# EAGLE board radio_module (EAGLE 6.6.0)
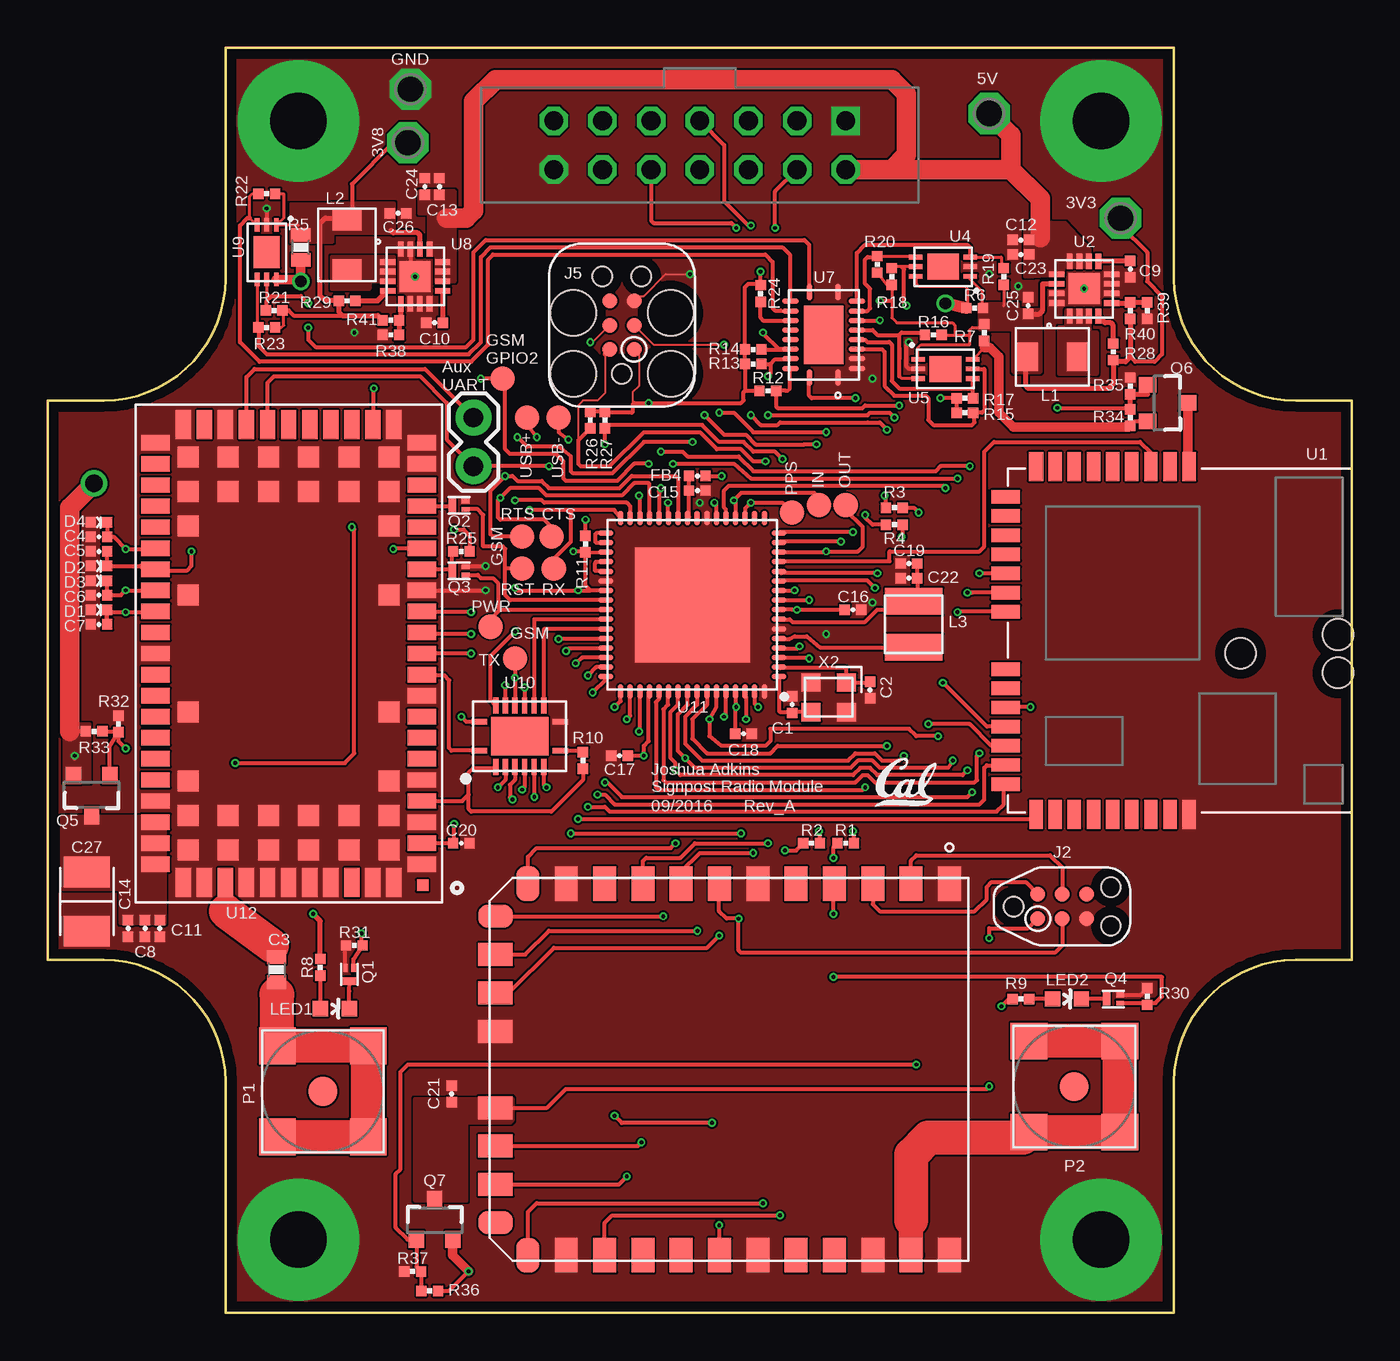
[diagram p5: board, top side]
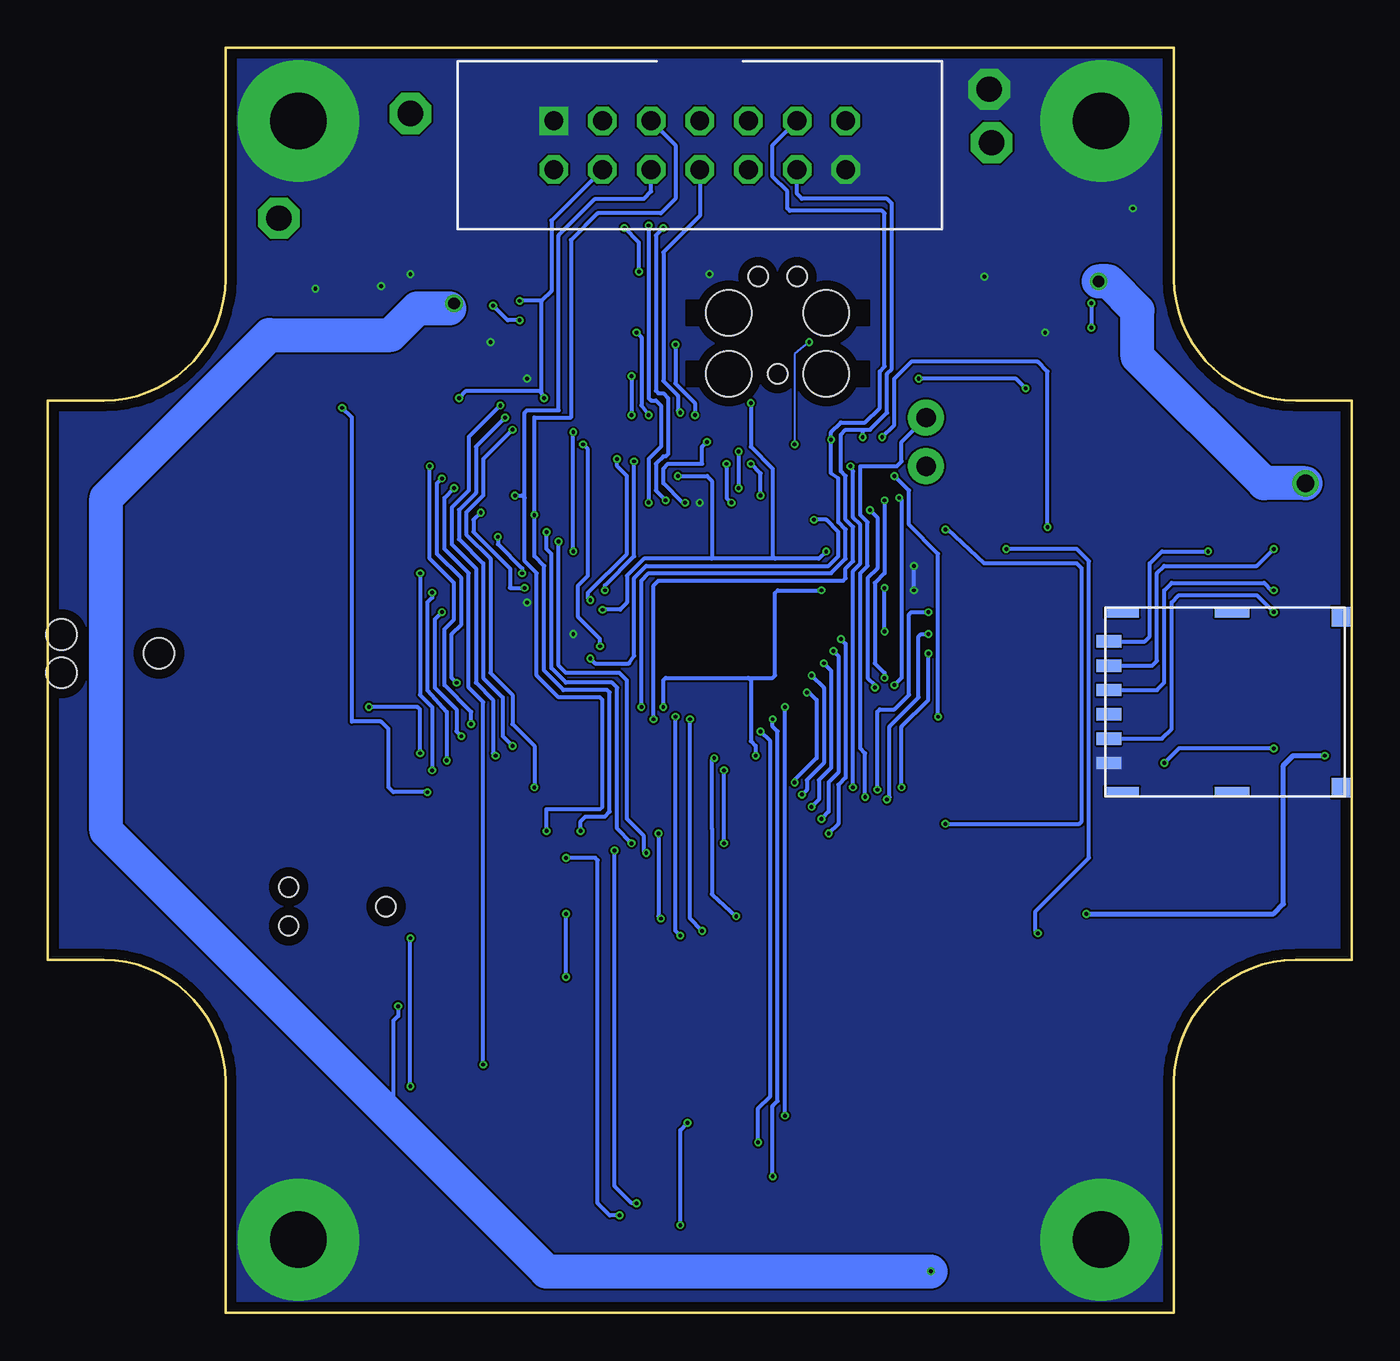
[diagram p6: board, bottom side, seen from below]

Size 68.07 x 66.04 mm. Coordinates in mm from the lower left corner, seen from the top.
Outline: 9.27,66.04 58.8,66.04 58.8,53.98 arc90 65.15,47.62 68.07,47.62 68.07,18.41 65.15,18.41 arc90 58.8,12.07 58.8,0 9.27,0 9.27,12.07 arc90 2.92,18.41 0,18.41 0,47.62 2.92,47.62 arc90 9.27,53.98 9.27,66.04
Copper layers (1*16): Top 0.0178mm / dielectric 59mil / Bottom 0.0178mm
Design rules "quickturn_co_kr_1oz *": minimum track width 4mil, minimum drill 0.200659375mm, track to track 4mil, track to pad 4mil, pad to pad 4mil, via to via 4mil, smd to smd 4mil, copper to edge 20mil, drill to drill 16mil, minimum pad ring 8mil, minimum via ring 4mil, stop-mask expansion 3mil, vias tented up to drill 50mil, thermal gap 10mil

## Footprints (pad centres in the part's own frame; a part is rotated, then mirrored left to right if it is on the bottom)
0402_CAP = smd 0.536 x 0.546: 1 -0.433,0; 2 0.433,0
0603_CAP = smd 0.7 x 1: 1 -0.65,0; 2 0.65,0
1210_CAP = smd 2.4 x 1.6: 1 0,1.55; 2 0,-1.55
0402_DIODE = smd 0.536 x 0.546: ANODE -0.433,0; CATHODE 0.433,0
MODULE_GENERIC = drill 0.991 square: 1 7.62,29.21 | drill 0.991 octagon: 2 7.62,26.67; 3 5.08,29.21; 4 5.08,26.67; 5 2.54,29.21; 6 2.54,26.67; 7 0,29.21; 8 0,26.67; 9 -2.54,29.21; 10 -2.54,26.67; 11 -5.08,29.21; 12 -5.08,26.67; 13 -7.62,29.21; 14 -7.62,26.67
TC2030-IDC-NL = smd 0.787 x 0.787: 1 -1.27,-0.635; 2 -1.27,0.635; 3 0,-0.635; 4 0,0.635; 5 1.27,-0.635; 6 1.27,0.635 | hole 1.016: -2.54,0; 2.54,1.016; 2.54,-1.016
WURTH_NANO_SIM = smd 0.65 x 1.3: C1 -1.905,6.07; C2 0.635,6.07; C3 1.905,6.07; C5 -3.175,6.07; C6 -0.635,6.07; C7 3.175,6.07 | smd 1.03 x 1: P$8 -4.465,-6.07; P$9 4.465,-6.07 | smd 0.48 x 1.8: P$10 -4.66,-0.35; P$11 4.66,-0.35; P$12 -4.66,5.4; P$13 4.66,5.4
TC2030-IDC = smd 0.787 x 0.787: 1 -1.27,-0.635; 2 -1.27,0.635; 3 0,-0.635; 4 0,0.635; 5 1.27,-0.635; 6 1.27,0.635 | hole 2.375: -2.54,2.54; 0.635,2.54; 0.635,-2.54; -2.54,-2.54 | hole 1.016: -2.54,0; 2.54,1.016; 2.54,-1.016
1X02 = drill 1.016 pad 1.88: 1 0,0; 2 2.54,0
IHL-1212BZ-11 = smd 1.2 x 1.5: P$1 -1.35,0; P$2 1.35,0
1212 = smd 1.4 x 3: P$1 -1.2,0; P$2 1.2,0
LED-0603 = smd 0.8 x 0.8: A 0,-0.75; C 0,0.75
SMA-J/PCB = smd 1.52 x 1.52: 1 0,0 | smd 1.91 x 1.91: 2 -2.375,-2.375; 3 2.375,-2.375; 4 2.375,2.375; 5 -2.375,2.375
XFDFN-3 = smd 0.4 x 0.7: D 0.35,0 | smd 0.4 x 0.25: G -0.35,0.215; S -0.35,-0.215
SOT23-3 = smd 0.8 x 0.9: 1 -0.95,-1; 2 0.95,-1; 3 0,1.1
0402_RES = smd 0.536 x 0.546: 1 -0.433,0; 2 0.433,0
0603-RES = smd 0.7 x 1: 1 -0.65,0; 2 0.65,0
B1,27 = smd 1.27 x 1.27: TP 0,0
P1-13 = drill 1.321 pad 2.159 octagon: TP 0,0
NUCLEUM = smd 0.7 x 1.5: 1 8.481,-0.109; 2 9.481,-0.109; 3 10.481,-0.109; 4 11.481,-0.109; 5 12.481,-0.109; 6 13.481,-0.109; 7 14.481,-0.109; 8 15.481,-0.109; 24 16.481,18.049; 25 15.481,18.049; 26 14.481,18.049; 27 13.481,18.049; 28 12.481,18.049; 29 11.481,18.049; 30 10.481,18.049; 31 9.481,18.049; 32 8.481,18.049 | smd 0.754 x 1.5: 9 16.481,-0.109 | smd 1.5 x 0.7: 10 18.06,1.47; 11 18.06,2.47; 12 18.06,3.47; 13 18.06,4.47; 14 18.06,5.47; 15 18.06,6.47; 16 18.06,7.47; 17 18.06,10.47; 18 18.06,11.47; 19 18.06,12.47; 20 18.06,13.47; 21 18.06,14.47; 22 18.06,15.47; 23 18.06,16.47 | hole 1.6: 0.72,8.66; 0.72,10.66; 5.8,9.64
TQFN-16/3MM = smd 0.3 x 0.8: 1 -0.75,-1.43; 2 -0.25,-1.43; 3 0.25,-1.43; 4 0.75,-1.43; 9 0.75,1.43; 10 0.25,1.43; 11 -0.25,1.43; 12 -0.75,1.43 | smd 0.8 x 0.3: 5 1.43,-0.75; 6 1.43,-0.25; 7 1.43,0.25; 8 1.43,0.75; 13 -1.43,0.75; 14 -1.43,0.25; 15 -1.43,-0.25; 16 -1.43,-0.75 | smd 1.63 x 1.63: GND 0,0
DFN-6-2MMX3MM = smd 0.25 x 0.7: 1 -0.5,-1.425; 2 0,-1.425; 3 0.5,-1.425; 4 0.5,1.425; 5 0,1.425; 6 -0.5,1.425 | smd 1.35 x 1.65: NC 0,0
IM880_MODULE = smd 1.8 x 1.2: 1 -9.7,11; 2 -9.7,9; 3 -9.7,7; 4 -9.7,5; 5 -9.7,3; 6 -9.7,1; 7 -9.7,-1; 8 -9.7,-3; 9 -9.7,-5; 10 -9.7,-7; 11 -9.7,-9; 12 -9.7,-11; 21 9.7,-11; 22 9.7,-9; 23 9.7,-7; 24 9.7,-5; 25 9.7,-3; 26 9.7,-1; 27 9.7,1; 28 9.7,3; 29 9.7,5; 30 9.7,7; 31 9.7,9; 32 9.7,11 | smd 1.2 x 1.8: 13 -8,-12.7; 14 -6,-12.7; 15 -4,-12.7; 16 -2,-12.7; 17 2,-12.7; 18 4,-12.7; 19 6,-12.7; 20 8,-12.7
QFN-N20 = smd 0.85 x 0.28: 1 -2.23,-0.75; 10 2.23,-0.75; 11 2.23,0.75; 20 -2.23,0.75 | smd 0.28 x 0.85: 2 -1.75,-1.73; 3 -1.25,-1.73; 4 -0.75,-1.73; 5 -0.25,-1.73; 6 0.25,-1.73; 7 0.75,-1.73; 8 1.25,-1.73; 9 1.75,-1.73; 12 1.75,1.73; 13 1.25,1.73; 14 0.75,1.73; 15 0.25,1.73; 16 -0.25,1.73; 17 -0.75,1.73; 18 -1.25,1.73; 19 -1.75,1.73 | smd 3.05 x 2.05: P$22 0,0
R-PVQFN-N16 = smd 0.825 x 0.28: 1 -2.112,-0.75; 8 2.112,-0.75; 9 2.112,0.75; 16 -2.112,0.75 | smd 0.28 x 0.825: 2 -1.25,-1.613; 3 -0.75,-1.613; 4 -0.25,-1.613; 5 0.25,-1.613; 6 0.75,-1.613; 7 1.25,-1.613; 10 1.25,1.613; 11 0.75,1.613; 12 0.25,1.613; 13 -0.25,1.613; 14 -0.75,1.613; 15 -1.25,1.613 | smd 3 x 2: THERMAL 0,0
QFN-64-9MM = smd 0.75 x 0.28: 1 -4.525,3.75; 2 -4.525,3.25; 3 -4.525,2.75; 4 -4.525,2.25; 5 -4.525,1.75; 6 -4.525,1.25; 7 -4.525,0.75; 8 -4.525,0.25; 9 -4.525,-0.25; 10 -4.525,-0.75; 11 -4.525,-1.25; 12 -4.525,-1.75; 13 -4.525,-2.25; 14 -4.525,-2.75; 15 -4.525,-3.25; 16 -4.525,-3.75; 33 4.525,-3.75; 34 4.525,-3.25; 35 4.525,-2.75; 36 4.525,-2.25; 37 4.525,-1.75; 38 4.525,-1.25; 39 4.525,-0.75; 40 4.525,-0.25; 41 4.525,0.25; 42 4.525,0.75; 43 4.525,1.25; 44 4.525,1.75; 45 4.525,2.25; 46 4.525,2.75; 47 4.525,3.25; 48 4.525,3.75 | smd 0.28 x 0.75: 17 -3.75,-4.525; 18 -3.25,-4.525; 19 -2.75,-4.525; 20 -2.25,-4.525; 21 -1.75,-4.525; 22 -1.25,-4.525; 23 -0.75,-4.525; 24 -0.25,-4.525; 25 0.25,-4.525; 26 0.75,-4.525; 27 1.25,-4.525; 28 1.75,-4.525; 29 2.25,-4.525; 30 2.75,-4.525; 31 3.25,-4.525; 32 3.75,-4.525; 49 3.75,4.525; 50 3.25,4.525; 51 2.75,4.525; 52 2.25,4.525; 53 1.75,4.525; 54 1.25,4.525; 55 0.75,4.525; 56 0.25,4.525; 57 -0.25,4.525; 58 -0.75,4.525; 59 -1.25,4.525; 60 -1.75,4.525; 61 -2.25,4.525; 62 -2.75,4.525; 63 -3.25,4.525; 64 -3.75,4.525 | smd 6 x 6: GND 0,0
UBLOX_SARA_G3 = smd 0.6 x 0.6: 1IND -12.1,-7 | smd 1.1 x 1.1: P65 -10.25,-5.25; P66 -10.25,-3.15; P67 -10.25,-1.05; P68 -10.25,1.05; P69 -10.25,3.15; P70 -10.25,5.25; P71 -8.45,-5.25; P72 -8.45,-3.15; P73 -8.45,-1.05; P74 -8.45,1.05; P75 -8.45,3.15; P76 -8.45,5.25; P77 -6.65,-5.25; P78 -6.65,5.25; P79 -3.05,-5.25; P80 -3.05,5.25; P81 3.05,-5.25; P82 3.05,5.25; P83 6.65,-5.25; P84 6.65,5.25; P85 8.45,-5.25; P86 8.45,-3.15; P87 8.45,-1.05; P88 8.45,1.05; P89 8.45,3.15; P90 8.45,5.25; P91 10.25,-5.25; P92 10.25,-3.15; P93 10.25,-1.05; P94 10.25,1.05; P95 10.25,3.15; P96 10.25,5.25 | smd 0.8 x 1.5: P$1 -11,-6.95; P$2 -9.9,-6.95; P$3 -8.8,-6.95; P$4 -7.7,-6.95; P$5 -6.6,-6.95; P$6 -5.5,-6.95; P$7 -4.4,-6.95; P$8 -3.3,-6.95; P$9 -2.2,-6.95; P$10 -1.1,-6.95; P$11 0,-6.95; P$12 1.1,-6.95; P$13 2.2,-6.95; P$14 3.3,-6.95; P$15 4.4,-6.95; P$16 5.5,-6.95; P$17 6.6,-6.95; P$18 7.7,-6.95; P$19 8.8,-6.95; P$20 9.9,-6.95; P$21 11,-6.95; P$33 11,6.95; P$34 9.9,6.95; P$35 8.8,6.95; P$36 7.7,6.95; P$37 6.6,6.95; P$38 5.5,6.95; P$39 4.4,6.95; P$40 3.3,6.95; P$41 2.2,6.95; P$42 1.1,6.95; P$43 0,6.95; P$44 -1.1,6.95; P$45 -2.2,6.95; P$46 -3.3,6.95; P$47 -4.4,6.95; P$48 -5.5,6.95; P$49 -6.6,6.95; P$50 -7.7,6.95; P$51 -8.8,6.95; P$52 -9.9,6.95; P$53 -11,6.95 | smd 1.5 x 0.8: P$22 11.95,-5.5; P$23 11.95,-4.4; P$24 11.95,-3.3; P$25 11.95,-2.2; P$26 11.95,-1.1; P$27 11.95,0; P$28 11.95,1.1; P$29 11.95,2.2; P$30 11.95,3.3; P$31 11.95,4.4; P$32 11.95,5.5; P$54 -11.95,5.5; P$55 -11.95,4.4; P$56 -11.95,3.3; P$57 -11.95,2.2; P$58 -11.95,1.1; P$59 -11.95,0; P$60 -11.95,-1.1; P$61 -11.95,-2.2; P$62 -11.95,-3.3; P$63 -11.95,-4.4; P$64 -11.95,-5.5
FHXXX = smd 1 x 0.95: 1 -0.925,-0.775; 2 0.925,-0.775; 3 0.925,0.775; 4 -0.925,0.775

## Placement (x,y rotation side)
C1  8pF  [0402_CAP]  38.86,31.75 90 top
C2  8pF  [0402_CAP]  42.93,32.51 270 top
C3  33pF  [0603_CAP]  11.94,17.91 270 top
C4  47pF  [0402_CAP]  2.67,40.51 180 top
C5  47pF  [0402_CAP]  2.67,39.75 180 top
C6  47pF  [0402_CAP]  2.67,37.47 180 top
C7  47pF  [0402_CAP]  2.67,35.94 180 top
C8  56pF  [0402_CAP]  5.08,20.07 270 top
C9  3.3nF  [0402_CAP]  56.52,54.48 90 top
C10  3.3nF  [0402_CAP]  20.19,51.69 0 top
C11  10nF  [0402_CAP]  5.84,20.07 270 top
C12  0.1uF  [0402_CAP]  50.8,56.01 180 top
C13  0.1uF  [0402_CAP]  20.45,58.8 90 top
C14  100nF  [0402_CAP]  4.19,20.07 270 top
C15  100nF  [0402_CAP]  33.91,42.93 0 top
C16  100nF  [0402_CAP]  42.04,36.7 0 top
C17  100nF  [0402_CAP]  29.85,29.08 180 top
C18  100nF  [0402_CAP]  36.32,30.23 0 top
C19  100nF  [0402_CAP]  44.96,39.12 180 top
C20  100nF  [0402_CAP]  21.59,24.51 0 top
C21  1uF  [0402_CAP]  21.08,11.43 90 top
C22  4.7uF  [0402_CAP]  44.96,38.35 180 top
C23  10uF  [0402_CAP]  50.8,55.24 180 top
C24  10uF  [0402_CAP]  19.68,58.8 90 top
C25  22uF  [0402_CAP]  51.18,52.58 270 top
C26  22uF  [0402_CAP]  18.29,57.4 180 top
C27  220uF  [1210_CAP]  2.03,21.46 0 top
D1  14V  [0402_DIODE]  2.67,36.7 0 top
D2  [0402_DIODE]  2.67,38.99 0 top
D3  [0402_DIODE]  2.67,38.23 0 top
D4  [0402_DIODE]  2.67,41.27 0 top
FB4  1.5k  [0402_CAP]  33.91,43.69 0 top
J1  MODULE_GENERIC  [MODULE_GENERIC]  34.04,33.02 0 top
J2  TC2030-JLINK-NL  [TC2030-IDC-NL]  52.96,21.21 0 top
J4  NANO_SIM  [WURTH_NANO_SIM]  6.6,31.88 90 bottom
J5  TC2030-JLINK-L  [TC2030-IDC]  29.97,51.56 90 top
JP1  [1X02]  22.22,44.2 90 top
L1  2.2uH  [IHL-1212BZ-11]  52.45,49.91 180 top
L2  2.2uH  [IHL-1212BZ-11]  15.62,55.75 90 top
L3  22uH  [1212]  45.21,35.94 270 top
LED1  LED0603  [LED-0603]  14.99,15.88 270 top
LED2  LED0603  [LED-0603]  53.21,16.38 270 top
P1  MOLEX_73251-135X  [SMA-J/PCB]  14.35,11.56 0 top
P2  MOLEX_73251-135X  [SMA-J/PCB]  53.59,11.81 180 top
Q1  MOSFET-NCHANNELXFDN-3  [XFDFN-3]  15.75,17.65 270 top
Q2  MOSFET-NCHANNELXFDN-3  [XFDFN-3]  21.46,42.16 180 top
Q3  MOSFET-NCHANNELXFDN-3  [XFDFN-3]  21.46,38.73 180 top
Q4  MOSFET-NCHANNELXFDN-3  [XFDFN-3]  55.63,16.38 180 top
Q5  SI223DDS  [SOT23-3]  2.29,27.05 180 top
Q6  SI223DDS  [SOT23-3]  58.42,47.5 270 top
Q7  SI223DDS  [SOT23-3]  20.19,4.83 0 top
R1  0  [0402_RES]  41.66,24.51 0 top
R2  0  [0402_RES]  39.88,24.51 0 top
R3  0  [0402_RES]  44.2,42.04 180 top
R4  0  [0402_RES]  44.2,41.15 180 top
R5  0.015  [0603-RES]  13.21,55.63 90 top
R6  0.43  [0402_RES]  48.39,52.45 0 top
R7  3.32  [0402_RES]  48.9,51.18 90 top
R8  1k  [0402_RES]  14.22,18.03 90 top
R9  1k  [0402_RES]  50.8,16.38 180 top
R10  10k  [0402_RES]  27.94,28.83 270 top
R11  10k  [0402_RES]  28.07,40.13 270 top
R12  10k  [0402_RES]  37.59,48.13 0 top
R13  10k  [0402_RES]  36.83,49.53 0 top
R14  10k  [0402_RES]  36.83,50.29 0 top
R15  10k  [0402_RES]  47.88,46.99 180 top
R16  10k  [0402_RES]  46.23,51.05 0 top
R17  10k  [0402_RES]  47.88,47.75 180 top
R18  10k  [0402_RES]  44.07,54.1 270 top
R19  10k  [0402_RES]  49.91,54.1 270 top
R20  10k  [0402_RES]  43.31,54.74 270 top
R21  10k  [0402_RES]  11.81,52.32 0 top
R22  10k  [0402_RES]  11.43,58.42 0 top
R23  10k  [0402_RES]  11.43,51.44 0 top
R24  10k  [0402_RES]  37.21,53.21 270 top
R25  100k  [0402_RES]  21.59,39.75 0 top
R26  100k  [0402_RES]  28.32,46.61 90 top
R27  100k  [0402_RES]  29.08,46.61 90 top
R28  100k  [0402_RES]  55.63,50.16 270 top
R29  100k  [0402_RES]  15.62,52.83 180 top
R30  100k  [0402_RES]  57.4,16.51 270 top
R31  100k  [0402_RES]  16,19.18 0 top
R32  100k  [0402_RES]  3.68,30.73 270 top
R33  100k  [0402_RES]  2.41,30.35 180 top
R34  100k  [0402_RES]  56.52,46.74 270 top
R35  100k  [0402_RES]  56.52,48.39 270 top
R36  100k  [0402_RES]  19.94,1.14 0 top
R37  100k  [0402_RES]  19.05,2.16 0 top
R38  200k  [0402_RES]  17.91,51.05 0 top
R39  240k  [0402_RES]  57.4,52.32 90 top
R40  750k  [0402_RES]  56.52,52.32 270 top
R41  750k  [0402_RES]  17.91,51.82 180 top
TP1  TPB1,27  [B1,27]  41.66,42.16 0 top
TP2  TPB1,27  [B1,27]  38.86,41.78 0 top
TP3  TPB1,27  [B1,27]  40.26,42.16 0 top
TP4  TPB1,27  [B1,27]  26.67,46.74 0 top
TP5  TPB1,27  [B1,27]  25.02,46.74 0 top
TP6  TPB1,27  [B1,27]  23.11,35.81 0 top
TP7  TPB1,27  [B1,27]  24.77,38.86 0 top
TP8  TPB1,27  [B1,27]  26.42,38.86 0 top
TP9  TPB1,27  [B1,27]  24.38,34.16 0 top
TP10  TPB1,27  [B1,27]  23.75,48.77 0 top
TP11  TPB1,27  [B1,27]  26.29,40.51 0 top
TP12  TPB1,27  [B1,27]  24.77,40.51 0 top
TP14  PTR1PAD1-13  [P1-13]  18.8,61.09 0 top
TP15  PTR1PAD1-13  [P1-13]  18.92,63.88 0 top
TP16  PTR1PAD1-13  [P1-13]  49.15,62.61 0 top
TP17  PTR1PAD1-13  [P1-13]  56.01,57.15 0 top
U1  NUCLEUM  [NUCLEUM]  68.07,44.07 180 top
U2  TLV62130  [TQFN-16/3MM]  54.1,53.47 0 top
U4  LTC2941  [DFN-6-2MMX3MM]  46.74,54.61 90 top
U5  LTC2941  [DFN-6-2MMX3MM]  46.86,49.28 270 top
U6  IM880_MODULE  [IM880_MODULE]  36.07,12.7 270 top
U7  PCA9544AQFN-N20  [QFN-N20]  40.51,51.05 90 top
U8  TLV62130  [TQFN-16/3MM]  19.18,54.1 270 top
U9  LTC2941  [DFN-6-2MMX3MM]  11.43,55.37 180 top
U10  TXB0106  [R-PVQFN-N16]  24.64,30.1 0 top
U11  SAM4LC8BA  [QFN-64-9MM]  33.66,36.96 180 top
U12  UBLOX_SARA_G350  [UBLOX_SARA_G3]  12.57,34.42 90 top
U$1  UCB_CAL100MIL  [UCB_CAL_100MIL]  43.18,26.42 0 top
X2  16 MHz  [FHXXX]  40.77,32.13 180 top

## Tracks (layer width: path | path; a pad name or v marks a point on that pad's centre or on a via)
3V3  (via drill 0.2)
  Top 0.102: J5.1 30.86,50.04 30.86,48.39 30.53,48.06 30.53,47.42
  Top 0.152: R7.2 48.72,51.44 48.26,51.44 48.13,51.31 48.13,51.05 | U4.1 48.16,53.95 48.77,53.34 48.77,52.45 R6.2 | R16.2 47.37,51.05 | 47.37,51.05 48.13,51.05 | U5.1 45.44,50.39 45.59,50.55 48.13,50.55 48.13,51.05 | R19.2 49.91,52.58 | R20.2 43.82,53.67 R18.2 44.07,52.83 44.07,51.94 44.32,51.69 47.24,51.69 47.37,51.56 47.37,51.05
  Top 0.203: R17.2 R15.2 | R17.2 47.37,47.68 | U11.35 29.1,39.68 R11.2 | U11.39 28.32,37.72 | 28.32,37.72 28.07,37.97 R11.2 | v43.43,52.83 44.07,52.83 | 39.75,48.9 U7.20 39.75,48.56 39.75,47.88 39.88,47.75 v42.16,47.75 | 36.4,48.13 R13.1 R14.1 36.4,53.54 36.58,53.72 37.14,53.72 R24.1 v37.21,54.36 | 36.4,48.13 R12.1 | U11.52 31.37,32.4 31.37,29.84 31.11,29.59 v31.11,29.08 C17.1 | U11.61 35.91,31.79 v35.94,31.62 35.89,31.7 C18.1 | 28.32,37.72 v27.69,37.72 24.51,37.72 v24.38,37.85 | U11.8 38.87,36.71 38.87,36.7 v39.12,36.7 C16.1 | R17.2 v46.61,47.75 | U10.15 23.11,31.99 23.11,34.29 v24.38,35.56 | FB4.2 v35.18,43.69 | R11.2 28.02,39.75 v27.43,39.75 | R26.2 R27.2 29.13,46.99 30.48,46.99 30.53,47.04 30.53,47.42 30.61,47.5 v31.37,47.5 36.2,47.5 36.32,47.62 36.32,48.06 36.4,48.13 | v37.97,56.64 37.97,58.55 J1.4 | TP17.TP 56.01,56.77 57.4,55.37 57.4,53.85 58.17,53.09 58.17,50.04 57.79,49.66 56.77,49.66 56.52,49.91
  Top 0.254: C25.2 51.76,52.15 51.94,52.32 51.94,53.72 U2.14 | L1.P$2 51.05,49.86 51.05,48.39 51.18,48.26 55.37,48.26 55.63,48.51 R28.2 55.7,49.66 56.26,49.66 56.52,49.91 R40.2
  Bottom 0.203: J1.4 41.78,57.02 41.78,53.34 42.29,52.83 | 42.29,52.83 v43.43,52.83 | v42.16,47.75 42.29,48.01 | 42.29,48.01 42.29,52.83 | v35.94,31.62 35.94,33.02 35.81,33.15 31.5,33.15 | 31.5,33.15 31.37,33.02 31.37,29.84 31.11,29.59 v31.11,29.08 | 31.5,33.15 30.23,33.15 30.1,33.27 30.1,37.59 29.97,37.72 v27.69,37.72 | v46.61,47.75 46.23,48.13 42.42,48.13 42.29,48.01 | v24.38,35.56 v24.38,37.85 | v27.43,39.75 27.81,39.37 30.1,39.37 | 30.1,39.37 33.4,39.37 | 33.4,39.37 36.96,39.37 37.85,38.48 37.85,37.08 38.18,36.75 U11.8 v39.12,36.7 | v35.18,43.69 33.66,43.69 33.4,43.43 33.4,39.37 | v31.37,47.5 31.37,45.21 30.23,44.07 30.23,39.5 30.1,39.37 | v37.21,54.36 37.21,55.88 v37.97,56.64
  pour Top (no thermals): 51.82,49.15 51.82,52.32 50.42,52.32 50.42,49.15
  pour Top (no thermals): 50.67,51.31 48.64,51.31 48.64,52.7 50.67,52.7
3V8
  Top 0.152: 13.08,56.77 13.05,56.8 U9.1 11.99,56.86 12.32,57.15 12.32,58.42 R22.2 | R23.2 12.19,51.44 12.32,51.56 12.32,52.15 R21.2
  Top 0.203: R21.2 12.57,52.32 12.83,52.07 15.37,52.07 | TP14.TP 18.03,61.09 15.88,58.93 15.88,57.36 L2.P$2
  Top 0.254: L2.P$2 15.57,57.15 14.48,57.15 14.22,56.9 14.22,53.09 14.48,52.83 R29.2 15.19,52.25 15.37,52.07 17.22,52.07 R41.2 | U8.14 19.43,56.27 19.3,56.39 18.03,56.39 17.91,56.52
  pour Top (no thermals): 14.86,57.91 18.03,57.91 18.03,56.39 14.86,56.39
  pour Top (no thermals): 12.7,55.88 12.7,57.91 14.86,57.91 14.86,55.88
3V8SWOUT
  pour Top (no thermals): 14.86,55.12 18.03,55.12 18.03,53.85 16.76,53.85 16.76,53.47 14.86,53.47
3VSWOUT
  pour Top (no thermals): 52.83,49.02 52.83,51.44 53.21,51.44 53.21,52.32 54.36,52.32 54.36,51.18 54.74,51.18 54.74,49.02
5V
  Top 0.254: U2.10
  Top 1.016: 50.29,59.69 J1.2 44.07,59.69 44.83,60.45 44.83,63.63 44.07,64.39 23.37,64.39 22.22,63.25 22.22,57.53 21.84,57.15 20.83,57.15 | 50.29,59.69 51.82,58.17 51.82,56.13 | 50.29,59.69 50.29,61.47 TP16.TP
  pour Top (no thermals): 54.36,54.61 52.96,54.61 52.96,54.23 51.05,54.1 51.05,56.9 53.09,56.9 54.36,55.5
  pour Top (no thermals): 19.94,55.24 19.94,57.4 19.43,57.4 19.43,58.55 21.21,58.55 21.21,53.85 20.32,53.85 20.32,55.24
!CONTROLLER_RESET  (via drill 0.2)
  Top 0.102: J5.3 31.62,50.55 v35.31,50.55
  Top 0.203: U11.4 38.22,34.67 39.12,34.67 v39.24,34.8 | v34.29,46.86 35.31,45.85 36.45,45.85 36.96,45.34 39.5,45.34 v40.13,45.34
  Bottom 0.203: v35.31,50.55 35.31,48.51 34.29,47.5 v34.29,46.86 | v39.24,34.8 39.24,35.18 40.39,36.32 40.39,37.97 39.88,38.48 39.88,45.09 v40.13,45.34
!GSM_RST
  Top 0.203: U11.40 24.13,37.21 23.88,37.47 23.88,38.86 | 23.88,38.86 23.88,39.88 23.75,40.01 22.73,40.01 22.73,41.66 22.44,41.95 Q2.G | TP7.TP 23.88,38.86
!IM880_RESET  (via drill 0.2)
  Top 0.203: U11.44 28.93,35.21 29.08,35.18 v26.67,35.18 | v27.3,25.02 v36.2,25.02 | 35.05,22.42 U6.7 35.05,22.38 35.05,20.96 35.43,20.57 v36.07,20.57 36.07,18.92 36.2,18.8 52.58,18.8 52.96,19.18 J2.3
  Bottom 0.203: v26.67,35.18 26.42,34.93 26.42,27.94 26.8,27.56 26.8,25.53 v27.3,25.02 | v36.2,25.02 36.2,20.7 v36.07,20.57
!NUCLEUM_RESET
  Top 0.203: U11.13 38.22,39.24 43.94,39.24 43.94,39.75 48.64,39.75 48.9,40.01 48.9,44.96 49.4,45.47 57.02,45.47 57.59,44.9 U1.3
CONTROLLER_BUCK/LDO_N  (via drill 0.2)
  Top 0.203: R11.1 v28.07,41.4 | U11.3 39.8,34.21 v39.75,34.16
  Bottom 0.203: v39.75,34.16 39.5,33.91 37.72,33.91 37.47,34.29 37.47,38.35 36.83,38.99 27.3,38.99 26.8,39.5 26.8,40.77 27.43,41.4 v28.07,41.4
CONTROLLER_SWDCLK  (via drill 0.2)
  Top 0.102: J5.4 28.45,50.67 v28.32,50.67
  Top 0.203: U11.9 v39.75,37.21 | v29.08,45.34 R27.1 29.26,46.36 34.16,46.36 35.05,45.47 36.32,45.47 36.83,44.96 37.97,44.96 v38.35,44.58
  Bottom 0.102: v28.32,50.67 29.08,50.04 v29.08,45.34
  Bottom 0.203: v39.75,37.21 39.88,37.34 39.88,37.59 37.85,39.62 37.85,43.69 38.35,44.2 v38.35,44.58
CONTROLLER_SWDIO  (via drill 0.2)
  Top 0.102: 29.08,50.04 29.08,48.01 28.7,47.62 27.94,47.62 27.69,47.37 27.69,45.54
  Top 0.203: U11.10 38.19,37.72 v38.99,37.72 | J5.2 29.08,50.04 | v37.47,44.45 36.83,44.45 36.2,45.09 34.93,45.09 34.04,45.97 31.11,45.97 29.34,44.2 27.81,44.2 27.69,44.32 27.69,45.54 R26.1
  Bottom 0.203: v38.99,37.72 38.99,37.97 37.47,39.5 v37.47,44.45
CONTROLLER_XIN
  Top 0.203: X2.3 38.77,31.36 C1.1 38.81,31.37 38.23,31.37 38.18,31.42 U11.1
CONTROLLER_XOUT
  Top 0.203: C2.1 42.89,32.91 X2.1 41.69,33.62 41.66,33.66 38.23,33.66 U11.2
GND  (via drill 0.2, 2.95 pad 6.35)
  Top 0.102: J5.5 30.86,53.09 31.11,53.09 32.26,54.23 v33.53,54.23
  Top 0.203: Q4.S 57.06,16.6 R30.1 | Q1.S 15.53,19.21 R31.1 | U8.15 18.93,54.35 U8.GND | v11.43,57.66 U9.2 | U5.2 44.96,49.28 44.83,49.4 44.83,50.55 v44.96,50.67 | U12.P$14 v22.86,37.72 | v22.86,38.99 22.82,38.95 Q3.S
  Top 0.254: 53.85,53.22 U2.GND 54.35,53.22
  Bottom 0.203: v22.86,37.72 v22.86,38.99
  other vias: 19.18,54.1 49.15,54.23 16,51.18 43.05,48.77 34.04,42.29 40.64,35.43 43.05,37.08 50.67,53.59 54.1,53.47 13.08,3.81 54.99,3.81 54.99,62.23 13.08,62.23
  pour Top (rank 2, no thermals): 58.8,66.04 58.8,54.23 arc90 65.53,47.62 68.07,47.62 68.07,18.41 67.95,18.41 67.95,18.29 65.41,18.29 arc90 58.8,11.68 58.8,0 9.27,0 9.27,11.68 arc90 3.43,18.41 0,18.41 0,47.62 3.05,47.62 arc90 9.14,53.72 9.27,53.72 9.27,66.04
  pour Bottom (no thermals): 9.27,0 9.27,12.19 arc90 3.05,18.41 0,18.41 0,47.62 2.79,47.62 arc90 9.27,54.1 9.27,66.04 58.8,66.04 58.8,53.98 arc90 65.15,47.62 68.07,47.62 68.07,18.41 65.15,18.41 arc90 58.8,12.07 58.8,0
GSM_3V8  (via drill 0.2, 0.61, 0.91)
  Top 0.152: 12.93,53.95 v13.21,53.85
  Top 0.203: R33.2 1.14,30.35
  Top 0.254: R8.2 14.22,20.45 v13.84,20.83 | v1.4,29.08 1.4,28.96
  Top 0.508: U9.6 12.93,53.95 13.08,53.92 v13.21,53.85 R5.1
  Top 1.016: 1.14,30.35 1.14,42.04 v2.41,43.31
  Bottom 0.254: v13.84,20.83 4.06,20.83 3.56,21.34 3.56,28.57 3.05,29.08 v1.4,29.08
  Bottom 1.778: v2.41,43.31 4.57,43.31 11.18,49.91 11.18,52.32 12.7,53.85 v13.21,53.85
  pour Top (no thermals): 0.89,27.69 0.89,30.73 2.16,30.73 2.16,30.61 2.16,27.69
GSM_AUX_RX
  Top 0.203: U11.43 29.11,35.69 25.91,35.69 25.89,35.67 U10.10
GSM_AUX_TX
  Top 0.203: U11.42 29.12,36.2 25.4,36.2 25.39,36.18 U10.11
GSM_CTS  (via drill 0.2)
  Top 0.203: U11.29 31.4,43.27 31.37,43.31 30.61,43.31 29.97,42.67 26.04,42.67 25.65,43.05 24.13,43.05 v23.62,42.55 23.5,42.42 23.5,41.53 23.62,41.4 25.91,41.4 26.29,41.02 TP11.TP | v23.88,32.77 23.88,31.72 U10.14
  Bottom 0.203: v23.62,42.55 23.5,42.42 23.5,33.15 v23.88,32.77
GSM_GATED
  pour Top (no thermals): 6.1,20.32 3.81,20.32 3.81,22.1 0.76,22.1 0.76,25.91 6.1,25.91
GSM_GAUGE_ALERT  (via drill 0.2)
  Top 0.152: U9.5 11.43,52.4 R21.1
  Top 0.203: 11.43,52.4 11.43,52.83 11.68,53.09 13.21,53.09 v13.59,52.7 | v13.59,51.44 13.59,50.8 13.97,50.42 21.84,50.42 22.22,50.8 22.22,55.37 22.86,56.01 39.5,56.01 39.75,55.75 39.75,53.3 U7.11
  Bottom 0.203: v13.59,52.7 v13.59,51.44
GSM_GAUGE_SCL
  Top 0.152: U9.3 10.89,56.8 10.54,57.15 10.54,58.29 10.67,58.42 R22.1
  Top 0.203: 10.54,57.15 10.41,57.15 10.03,56.77 10.03,50.67 11.05,49.66 22.1,49.66 22.99,50.55 22.99,54.99 23.24,55.24 37.47,55.24 37.85,54.86 37.85,52.45 37.97,52.32 38.26,52.32 U7.13
GSM_GAUGE_SDA
  Top 0.152: U9.4 10.93,51.5 R23.1
  Top 0.203: R23.1 11,50.47 11.43,50.04 21.97,50.04 22.61,50.67 22.61,55.12 23.11,55.63 38.35,55.63 38.74,55.24 38.74,53.01 U7.12 38.76,52.96
GSM_GPIO2  (via drill 0.2)
  Top 0.203: U12.P$23 17.02,46.41 v17.02,48.26 | U11.30 30.9,42.63 v30.86,42.67 | v31.37,44.32 30.61,44.32 29.72,43.43 27.05,43.43 26.92,43.56 26.92,44.45 26.54,44.83 24.13,44.83 23.88,45.09 23.88,48.51 23.62,48.77 v22.61,48.77 TP10.TP
  Bottom 0.203: v17.02,48.26 17.53,48.77 v22.61,48.77 | v30.86,42.67 30.86,43.81 v31.37,44.32
GSM_LED  (via drill 0.2)
  Top 0.203: Q1.G 15.96,18.45 R31.2 16.38,19.23 v16.38,19.81 | v18.03,39.88 18.07,39.92 U12.P$16
  Bottom 0.203: v16.38,19.81 16.51,19.94 16.51,20.96 13.72,23.75 13.72,39.24 14.35,39.88 v18.03,39.88
GSM_POWER
  Top 0.203: Q3.G 22.44,38.52 22.61,38.35 23.24,38.35 23.5,38.1 23.5,36.83 23.62,36.7 | 23.62,36.7 U11.41 | TP6.TP 23.11,36.2 23.62,36.7
GSM_POWER_GATE  (via drill 0.2)
  Top 0.203: Q5.1 3.24,29.6 R32.2 | R33.1 3.63,30.35 R32.2 | R32.2 3.68,29.84 v4.06,29.46 | v9.78,28.7 15.49,28.7 16,29.21 16,40.89 v15.88,41.02 | U11.22 34.91,42.14 v34.8,42.29 | v33.66,45.47 31.11,45.47 29.46,43.81 27.43,43.81 27.3,43.94 27.3,44.7 26.67,45.21 25.02,45.21 v24.51,45.72
  Bottom 0.203: v4.06,29.46 9.02,29.46 v9.78,28.7 | v15.88,41.02 15.88,49.15 16.38,49.66 22.99,49.66 23.88,48.77 23.88,46.36 v24.51,45.72 | v34.8,42.29 34.93,42.29 35.94,43.31 35.94,44.07 35.69,44.32 33.91,44.32 33.91,45.21 v33.66,45.47
GSM_RTS  (via drill 0.2)
  Top 0.203: U10.16 21.86,30.85 v21.59,31.12 | U11.26 32.91,43.55 32.77,43.69 30.48,43.69 29.85,43.05 26.16,43.05 25.78,43.43 24.51,43.43 24.26,43.69 v23.88,43.69 23.11,42.93 23.11,40.64 23.24,40.51 TP12.TP
  Bottom 0.203: v21.59,31.12 21.59,39.62 23.11,41.15 23.11,42.93 v23.88,43.69
GSM_RX  (via drill 0.2)
  Top 0.203: U11.32 29.57,41.91 27.43,41.91 | 27.43,41.91 v25.15,41.91 | v24.89,32.64 v24.89,32.63 U10.12 | TP8.TP 26.42,39.37 27.3,40.26 27.3,41.78 27.43,41.91
  Bottom 0.203: v25.15,41.91 24.77,41.53 24.77,38.86 25.27,38.35 25.27,33.15 24.89,32.77 v24.89,32.64
GSM_TX  (via drill 0.2)
  Top 0.203: U11.31 30.4,42.11 30.23,42.29 25.91,42.29 25.78,42.42 v24.38,42.42 | U10.13 24.39,33.02 v24.38,33.15 TP9.TP
  Bottom 0.203: v24.38,42.42 24.38,38.61 24.89,38.1 24.89,33.91 24.38,33.4 v24.38,33.15
IM880_3V3  (via drill 0.2, 0.61)
  Top 0.152: U4.6 45.31,53.75 45.47,53.59 47.88,53.59 48.01,53.47 48.01,52.5 R6.1
  Top 0.203: R36.2 20.95,1.14 v21.97,2.16 | R9.2 50.17,16.38 v49.78,16
  Top 0.508: Q7.2 21.14,2.99 v21.97,2.16
  Top 0.61: R6.1 v46.86,52.7
  Bottom 0.203: v49.78,16 49.78,15.49 50.04,15.24 50.04,10.92 50.42,10.54
  Bottom 1.016: 47.12,52.45 v46.86,52.7
  Bottom 1.778: 47.12,52.45 48.77,52.45 50.17,51.05 56.52,51.05 65.02,42.55 65.02,25.15 50.42,10.54 42.04,2.16 v21.97,2.16
IM880_BOOT  (via drill 0.2)
  Top 0.203: v29.59,31.62 29.9,31.94 U11.49 | v29.59,10.29 29.97,9.91 v34.67,9.91 | U6.26 35.07,4.56 v35.05,4.57
  Bottom 0.203: v29.59,10.29 v29.59,31.62 | v35.05,4.57 35.05,9.52 v34.67,9.91
IM880_CS  (via drill 0.2)
  Top 0.203: U6.15 24.07,16.7 26.42,19.05 34.42,19.05 v35.05,19.69 | v35.31,31.12 35.41,31.27 U11.60
  Bottom 0.203: v35.05,19.69 35.31,19.94 v35.31,31.12
IM880_GATED  (via drill 0.2)
  Top 0.203: U6.17 26.07,10.7 27.05,11.68 49.02,11.68 v49.15,11.81 | v49.15,19.56 49.15,20.07 51.18,20.07 J2.1
  Bottom 0.203: v49.15,11.81 v49.15,19.56
  pour Top (no thermals): 20.95,5.84 19.18,5.84 19.18,11.18 24.26,11.18 24.26,10.03 24.13,9.91 21.84,9.91 21.84,5.84
IM880_GAUGE_ALERT  (via drill 0.2)
  Top 0.152: U4.5 44.58,54.61 44.14,54.61 R18.1
  Top 0.203: U7.7 43.42,51.8 v43.43,51.82 | v44.83,52.58 44.7,52.7 44.7,54.48 44.58,54.61
  Bottom 0.203: v43.43,51.82 44.07,51.82 v44.83,52.58
IM880_GAUGE_SCL
  Top 0.152: U4.3 49.78,55.12 49.78,54.74 R19.1
  Top 0.203: U7.9 42.24,55.32 42.67,55.75 48.01,55.75 48.13,55.63 48.13,55.14 U4.3
IM880_GAUGE_SDA
  Top 0.152: R20.1 45.24,55.17 U4.4
  Top 0.203: U7.8 42.78,52.3 42.93,52.45 42.93,53.47 42.67,53.72 42.67,54.99 42.8,55.12 43.26,55.12 R20.1
IM880_INT1  (via drill 0.2)
  Top 0.203: U6.8 33.07,23.04 34.04,24 v36.83,24 | v41.4,40.26 38.23,40.26 U11.15
  Bottom 0.203: v36.83,24 36.96,24.13 36.96,24.89 37.85,25.78 37.85,33.02 38.23,33.4 41.02,33.4 41.4,33.78 v41.4,40.26
IM880_INT2  (via drill 0.2)
  Top 0.203: U6.9 31.07,23.57 31.24,23.75 33.02,23.75 33.78,24.51 v37.59,24.51 | v42.04,40.77 38.24,40.77 U11.16
  Bottom 0.203: v37.59,24.51 38.35,25.27 38.35,32.64 38.61,32.89 41.02,32.89 41.78,33.66 41.78,39.62 42.04,39.88 v42.04,40.77
IM880_NETWORK  (via drill 0.2)
  Top 0.203: 57.31,16.17 R30.2 | Q4.G 57.31,16.17 | 57.31,16.17 57.82,16.17 58.17,16.51 58.17,17.53 v41.02,17.53 | v41.02,20.83 41.02,22.35 U6.4
  Bottom 0.203: v41.02,17.53 v41.02,20.83
IM880_POWER_GATE  (via drill 0.2)
  Top 0.203: R36.1 19.48,1.17 R37.2 19.24,2.4 Q7.1 18.78,3.83 18.16,4.45 18.16,7.24 18.41,7.49 18.41,12.57 18.8,12.95 v45.34,12.95 | U11.21 35.41,41.94 35.31,42.04 35.31,42.93 35.56,43.18 46.74,43.18 v46.86,43.05
  Bottom 0.203: v45.34,12.95 45.34,31.88 46.1,32.64 46.1,38.61 47.37,39.88 47.37,42.55 v46.86,43.05
IM880_RX  (via drill 0.2)
  Top 0.203: v30.86,30.35 30.9,30.44 U11.51 | U6.18 30.8,8.7 v30.99,8.89
  Bottom 0.203: v30.86,30.35 30.35,29.84 30.35,11.3 30.99,10.67 v30.99,8.89
IM880_SWCLK
  Top 0.203: U6.2 45.07,23.61 45.34,23.88 52.32,23.88 52.96,23.24 J2.4
IM880_SWDIO
  Top 0.203: U6.3 43.07,21.32 43.43,20.96 48.39,20.96 49.02,21.59 49.02,22.23 49.28,22.48 51.05,22.48 J2.2
IM880_TX  (via drill 0.2)
  Top 0.203: v30.23,30.99 30.4,31.17 U11.50 | U6.19 29.81,6.7 v30.23,7.11
  Bottom 0.203: v30.23,7.11 30.23,10.8 29.97,11.05 29.97,30.35 30.23,30.61 v30.23,30.99
MISO  (via drill 0.2)
  Top 0.203: 32.89,32.42 U11.55 32.91,31.76 32.51,31.37 32.51,28.96 32.77,28.7 v32.77,28.32 33.02,28.07 42.04,28.07 42.42,28.45 42.93,28.45 43.31,28.07 47.75,28.07 v48.01,28.32 | U6.12 25.07,23.8 25.53,24.26 32.51,24.26 v32.77,24.51 | U1.14 48.78,38.6 v48.64,38.61
  Bottom 0.203: v32.77,24.51 v32.77,28.32 | v48.64,38.61 48.64,32.26 48.01,31.62 v48.01,28.32
MOD_IN  (via drill 0.2)
  Top 0.203: U11.20 35.91,42.33 v35.81,42.42 36.2,42.8 40.01,42.8 40.13,42.67 TP3.TP | J1.10 31.5,57.02 31.62,56.9 35.69,56.9 v35.94,56.64
  Bottom 0.203: v35.81,42.42 36.32,42.93 36.32,44.32 35.94,44.7 35.81,44.7 35.69,44.83 35.69,47.75 35.94,48.01 36.2,48.01 36.32,48.13 36.32,56.26 v35.94,56.64
MOD_OUT  (via drill 0.2)
  Top 0.203: v35.05,46.99 35.81,46.99 36.83,45.97 v40.64,45.97 | U11.14 40.56,39.71 v40.64,39.75 42.29,39.75 42.55,40.01 42.55,41.02 41.66,41.91 TP1.TP
  Bottom 0.203: J1.8 34.04,57.28 35.94,55.37 35.94,48.64 35.18,47.88 35.18,47.12 v35.05,46.99 | v40.64,39.75 v40.64,45.97
MOSI  (via drill 0.2)
  Top 0.203: U6.13 32.01,20.7 v32.13,20.7 | U11.56 33.41,31.75 32.89,31.24 32.89,29.34 v33.28,28.96 33.4,28.83 33.78,28.45 41.91,28.45 42.29,28.83 43.05,28.83 43.43,28.45 46.99,28.45 v47.24,28.83 | U1.15 48.27,37.6 v48.01,37.59
  Bottom 0.203: v32.13,20.7 33.4,21.84 33.4,25.27 33.41,25.28 33.41,28.83 v33.28,28.96 | v48.01,37.59 48.01,37.34 48.26,37.08 48.26,32.51 47.24,31.37 v47.24,28.83
N$1  (via drill 0.2)
  Top 0.203: D1.CATHODE 2.97,36.65 3.02,36.65 | U12.P$41 5.58,36.58 v4.06,36.58 3.05,36.58 C7.1 | 3.02,36.65 3.05,36.65 C7.1 | 3.02,36.65 C7.1
  Bottom 0.203: J4.C1 9.91,29.97 9.4,30.48 9.4,37.08 9.02,37.47 4.95,37.47 v4.06,36.58
N$2  (via drill 0.2)
  Top 0.203: D3.CATHODE C6.1 3.81,37.47 v4.06,37.72 U12.P$40
  Bottom 0.203: J4.C2 10.16,32.51 9.78,32.89 9.78,37.72 9.4,38.1 4.57,38.1 4.19,37.72 v4.06,37.72
N$3  (via drill 0.2)
  Top 0.203: C5.1 D2.CATHODE 4.83,38.99 5.08,38.73 5.54,38.73 | v7.49,39.75 7.49,38.99 7.24,38.73 5.54,38.73 | 5.54,38.73 U12.P$39
  Bottom 0.203: J4.C7 10.79,35.05 10.54,35.31 10.54,39.12 9.91,39.75 v7.49,39.75
N$4  (via drill 0.2)
  Top 0.203: D4.CATHODE C4.1 3.43,40.51 v4.06,39.88 5.58,39.88 U12.P$38
  Bottom 0.203: J4.C3 10.41,33.78 10.16,34.04 10.16,38.61 9.78,38.99 4.95,38.99 v4.06,39.88
N$5
  Top 0.203: U10.8 27.85,29.35 R10.1
N$6
  Top 0.203: U12.P$56 9.27,21.08 9.14,20.96 9.29,20.96 | 11.68,19.18 11.68,18.56 C3.1
  Top 1.778: 9.29,20.96 11.68,19.18
N$7
  Top 0.203: 11.94,16.64 C3.2
  Top 1.778: P1.2 P1.3 P1.4 P1.5 11.98,16.6 11.94,16.64
N$8
  Top 0.203: R8.1 14.22,15.89 LED1.A
N$9  (via drill 0.2)
  Top 0.203: U11.53 31.9,32.03 31.75,31.88 31.75,27.43 31.88,27.3 42.55,27.3 v42.67,27.43 | v36.7,46.86 37.21,46.36 38.1,46.36 38.23,46.48 42.8,46.48 43.43,46.48 v43.82,46.1 | v37.34,51.18 37.39,51.13 37.39,51.08 38.16,50.3 U7.17 38.77,50.29 R14.2
  Bottom 0.203: v37.34,51.18 37.08,50.93 37.08,47.37 v36.7,46.86 | v43.82,46.1 45.34,44.58 45.34,42.67 46.23,41.78 46.23,40.64 44.96,39.37 44.96,33.4 43.82,32.26 43.82,30.73 42.67,29.59 v42.67,27.43
N$10  (via drill 0.2)
  Top 0.203: U10.4 24.39,27.82 24.13,27.56 24.13,26.92 v24.26,26.8 | v22.1,35.43 19.61,35.43 U12.P$12
  Bottom 0.203: v24.26,26.8 24.13,26.92 24.13,30.61 22.61,32.13 22.61,35.31 22.48,35.43 v22.1,35.43
N$11  (via drill 0.2)
  Top 0.203: U10.5 24.89,27.43 v24.77,27.3 | v22.1,36.58 19.56,36.58 U12.P$13
  Bottom 0.203: v24.77,27.3 24.77,31.37 24.64,31.5 23.88,31.5 23.11,32.26 23.11,36.45 22.99,36.58 v22.1,36.58
N$12
  Top 0.203: R24.2 37.21,51.94 37.35,51.8 U7.14
N$13
  Top 0.203: LED1.C 15.74,16.78 Q1.D
N$14
  Top 0.203: U12.P$18 21.07,42.12 Q2.D
N$15  (via drill 0.2)
  Top 0.203: U12.P$2 C20.1 21.21,24.56 v21.21,25.53 | v21.21,40.89 21.72,40.89 22.02,40.59 R25.2
  Bottom 0.203: v21.21,25.53 14.22,25.53 14.1,25.65 14.1,38.86 14.35,39.12 19.18,39.12 21.08,40.89 v21.21,40.89
N$16
  Top 0.203: U12.P$15 21.03,38.82 Q3.D 21.11,39.71 R25.1
N$17  (via drill 0.2)
  Top 0.203: R3.1 45.21,42.04 v45.47,41.78 | v43.18,37.85 42.8,38.23 38.2,38.23 U11.11
  Bottom 0.203: v45.47,41.78 45.85,41.4 45.85,40.77 43.94,38.86 43.94,37.85 v43.18,37.85
N$18  (via drill 0.2)
  Top 0.203: R4.1 44.63,40.56 v44.58,40.51 | v43.31,38.61 38.28,38.61 U11.12
  Bottom 0.203: v44.58,40.51 44.58,40.13 43.31,38.86 v43.31,38.61
N$19
  Top 0.508: Q6.3 59.52,44.25 U1.1
N$20  (via drill 0.2)
  Top 0.203: U12.P$29 10.37,48.85 10.79,49.28 19.68,49.28 JP1.2 | U10.6 25.39,26.94 v25.4,26.92
  Bottom 0.203: v25.4,26.92 25.4,29.21 25.65,29.46 25.65,38.61 25.27,38.99 25.27,41.27 25.65,41.66 25.65,44.2 23.75,44.2 23.5,44.45 23.5,45.47 JP1.2
N$21  (via drill 0.2)
  Top 0.203: U12.P$28 11.47,48.56 11.81,48.9 19.43,48.9 20.83,47.5 20.83,45.59 JP1.1 v26.16,44.2 | U10.7 25.89,27.58 v26.04,27.43
  Bottom 0.203: v26.04,27.43 26.04,38.73 25.65,39.12 25.65,41.15 26.04,41.53 26.04,43.94 v26.16,44.2
N$22  (via drill 0.2)
  Top 0.203: U10.3 23.89,27.82 v23.5,27.43 | v22.1,34.42 U12.P$11
  Bottom 0.203: v23.5,27.43 23.5,30.61 22.1,32 v22.1,34.42
N$23
  Top 0.203: U12.P$10 19.57,33.27 20.7,33.27 20.95,33.02 20.95,29.46 21.07,29.35 U10.1
N$25  (via drill 0.2)
  Top 0.203: U6.23 29.07,4.68 29.46,5.08 v38.23,5.08 | v41.02,23.75 41.02,24.31 R1.1
  Bottom 0.203: v38.23,5.08 38.74,5.08 39.37,5.72 39.37,23.62 39.5,23.75 v41.02,23.75
N$26  (via drill 0.2)
  Top 0.203: U6.21 25.07,5.26 25.53,5.72 v37.34,5.72 | v38.48,24.13 39.06,24.13 R2.1
  Bottom 0.203: v38.48,24.13 38.48,6.6 37.59,5.72 v37.34,5.72
N$27
  Top 0.203: LED2.A R9.1
N$28
  Top 0.203: Q4.D LED2.C
N$29
  Top 1.27: U6.31 45.07,4.81 45.09,4.83
  Top 1.778: 45.09,4.83 45.09,8.25 45.97,9.14 50.93,9.14 P2.4 P2.5 P2.2 P2.3
N$33
  Top 0.203: U11.25 33.48,41.55 C15.1 FB4.1
N$34
  Top 0.254: C9.2 U2.9
N$36
  Top 0.254: R28.1 55.63,51.56 55.5,51.69 55.2,51.69 U2.4
N$37
  Top 0.254: U2.5 56.48,52.72 R40.1 R39.2
N$38
  Top 0.254: U8.9 20.61,51.71 C10.2
N$40
  Top 0.254: R29.1 17.23,52.83 U8.4
N$41
  Top 0.254: U8.5 18.43,51.9 R41.1 R38.2
N$44
  Top 0.203: U11.7 38.19,36.2 38.74,36.2 38.86,36.07 42.67,36.07 43.31,36.7 44.77,36.7 L3.P$1 45.39,37.32 C22.1 C19.1
N$52
  Top 0.203: U11.5 38.21,35.18 38.74,35.18 38.99,35.31 39.62,35.31 40.32,34.74 L3.P$2
N$53
  Top 0.203: U11.37 29.1,38.73 28.57,38.73 28.57,39.12 28.61,39.21 U11.36
N$54
  Top 0.203: U11.33 28.64,40.71 28.57,40.64 28.57,40.26 28.63,40.21 U11.34
NUCLEUM_3V3
  Top 0.152: R7.1 48.9,50.38 U5.6
  Top 0.203: R34.2 56.76,46.55 Q6.2
  Top 0.508: 48.9,50.38 49.19,50.38 49.66,49.91 49.66,46.99 50.42,46.23 56.44,46.23 R34.2
NUCLEUM_BOOT  (via drill 0.2)
  Top 0.203: U11.45 29.17,34.71 29.08,34.67 27.18,34.67 v27.05,34.54 | v27.69,25.78 51.35,25.78 U1.24
  Bottom 0.203: v27.05,34.54 26.8,34.29 26.8,28.19 27.3,27.69 27.3,26.16 v27.69,25.78
NUCLEUM_CS  (via drill 0.2)
  Top 0.203: v51.31,31.62 50.04,31.62 U1.19 | U11.54 32.39,32.41 32.39,31.75 32.13,31.5 32.13,27.81 32.26,27.69 42.16,27.69 42.55,28.07 42.8,28.07 43.18,27.69 48.39,27.69 48.51,27.81 48.51,29.08 v48.64,29.21
  Bottom 0.203: v48.64,29.21 48.64,31.5 48.77,31.62 v51.31,31.62
NUCLEUM_GAUGE_ALERT
  Top 0.203: U5.5 48.9,49.28 48.9,47.12 48.77,46.99 R15.1 48.39,46.91 48.39,46.48 48.26,46.36 46.23,46.36 45.97,46.61 45.97,47.75 45.85,47.88 44.2,47.88 43.69,48.39 43.69,50.16 43.55,50.3 U7.4
NUCLEUM_GAUGE_SCL
  Top 0.152: U5.3 44.57,48.78 44.45,48.9 | 45.67,51.18 R16.1
  Top 0.203: 44.45,48.9 44.45,49.78 | 44.45,49.78 44.45,51.05 44.58,51.18 45.67,51.18 | U7.6 43.06,51.3 43.31,51.05 44.45,51.05 44.45,49.78
NUCLEUM_GAUGE_SDA
  Top 0.203: R17.1 48.29,47.78 48.29,48.26 | 48.29,48.26 U5.4 | U7.5 42.67,50.8 42.8,50.67 43.94,50.68 44.07,50.55 44.07,48.64 44.45,48.26 48.29,48.26
NUCLEUM_INT1/RTS  (via drill 0.2, 0.2 pad 0.41)
  Top 0.203: U1.20 49.03,30.6 v46.74,32.89 | v32.64,44.32 35.81,44.32 36.7,43.56 v47.5,43.56 | U11.27 32.39,41.5 v32.39,42.29
  Bottom 0.203: v32.64,44.32 32.64,42.55 v32.39,42.29 | v46.74,32.89 46.99,33.15 46.99,35.43 46.48,35.94 46.48,38.35 47.75,39.62 47.75,43.31 v47.5,43.56
NUCLEUM_INT2/CTS  (via drill 0.2)
  Top 0.203: U1.21 49.27,29.6 48.13,30.73 v45.97,30.73 | v32,44.96 33.15,44.96 33.4,44.7 36.07,44.7 36.83,43.94 46.36,43.94 46.61,44.2 v48.13,44.2 | v32,43.05 31.9,42.9 U11.28
  Bottom 0.203: v45.97,30.73 45.97,31.37 47.37,32.77 47.37,35.69 46.86,36.2 46.86,38.1 48.13,39.37 v48.13,44.2 | v32,44.96 v32,43.05
NUCLEUM_POWER_GATE  (via drill 0.2)
  Top 0.203: U11.48 29.13,33.07 v28.45,32.38 | v29.08,27.69 29.21,27.69 29.97,26.92 48.01,26.92 v48.26,27.18 | v52.71,47.24 56.44,47.24 R34.1
  Top 0.254: R34.1 R35.2 57.41,47.95 Q6.1
  Bottom 0.203: v28.45,32.38 28.32,32.38 27.94,32 27.94,28.96 29.08,27.81 v29.08,27.69 | v48.26,27.18 50.04,27.18 50.29,27.43 50.29,30.48 50.67,30.86 52.2,30.86 52.2,46.74 v52.71,47.24
NUCLEUM_RX  (via drill 0.2)
  Top 0.203: U11.47 28.63,33.71 v28.19,33.27 | v28.7,27.05 29.08,27.05 29.59,26.54 48.64,26.54 48.9,26.8 48.9,28.45 49.02,28.57 49.99,28.57 U1.22
  Bottom 0.203: v28.19,33.27 27.56,32.64 27.56,28.7 28.45,27.81 28.45,27.3 v28.7,27.05
NUCLEUM_TX  (via drill 0.2)
  Top 0.203: U11.46 27.9,34.21 v27.56,33.91 | v28.19,26.42 29.08,26.42 29.34,26.16 49.53,26.16 49.91,26.54 49.91,27.5 U1.23
  Bottom 0.203: v27.56,33.91 27.18,33.53 27.18,28.45 27.81,27.81 27.81,26.8 v28.19,26.42
PPS  (via drill 0.2)
  Top 0.203: J1.7 35.31,60.96 35.31,58.04 36.58,56.77 v36.7,56.77 | U11.19 36.41,41.99 v36.7,42.29 38.35,42.29 TP2.TP
  Bottom 0.203: v36.7,56.77 36.7,47.75 36.58,47.62 36.32,47.62 36.07,47.37 36.07,45.21 36.7,44.58 v36.7,42.29
SCL  (via drill 0.2)
  Top 0.203: R2.2 40.31,25.09 v40.26,25.15 | R4.2 43.05,41.15 42.67,41.53 v42.67,41.66
  Bottom 0.203: J1.5 35.31,60.96 35.31,58.17 36.07,57.4 39.37,57.4 40.77,56.01 40.77,46.74 42.67,46.74 v42.67,41.66 42.67,39.5 42.16,38.99 42.16,33.53 41.15,32.51 38.86,32.51 38.74,32.38 38.74,26.16 38.99,25.91 40.01,25.91 40.26,25.65 v40.26,25.15
SCL_INTERNAL  (via drill 0.2)
  Top 0.203: U11.58 34.41,31.74 33.66,30.99 33.66,29.97 34.42,29.21 37.72,29.21 38.1,29.59 v43.82,29.59 | 37.64,48.95 v37.59,48.9 37.72,49.02 37.72,49.53 | v37.59,46.86 42.8,46.86 42.93,46.99 43.94,46.99 v44.2,46.74 | R13.2 37.72,49.53 | 37.72,49.53 37.97,49.78 38.76,49.78 U7.18
  Bottom 0.203: v37.59,48.9 v37.59,46.86 | v44.2,46.74 45.72,45.21 45.72,42.8 46.61,41.91 46.61,40.39 45.34,39.12 45.34,33.15 44.32,32.13 44.32,30.1 v43.82,29.59
SCLK  (via drill 0.2)
  Top 0.203: U6.14 24.92,18.7 26.16,19.94 v33.91,19.94 | U11.59 34.91,31.64 v34.54,30.99 34.54,30.1 35.18,29.59 37.47,29.59 37.72,29.84 37.72,30.48 44.96,30.48 45.34,30.1 v46.48,30.1 | U1.16 47.52,36.6 v47.5,36.58
  Bottom 0.203: v33.91,19.94 34.54,20.57 v34.54,30.99 | v47.5,36.58 47.88,36.2 47.88,32.64 46.74,31.5 46.74,30.35 v46.48,30.1
SDA  (via drill 0.2)
  Top 0.203: R1.2 42.09,25.09 v42.04,25.15 | R3.2 43.76,42.6 v43.69,42.67
  Bottom 0.203: J1.6 36.58,58.55 36.96,58.17 39.5,58.17 41.4,56.26 41.4,47.12 43.05,47.12 43.18,46.99 43.18,42.55 | v42.04,25.15 42.04,26.29 39.24,26.29 39.12,26.42 39.12,32 39.24,32.13 41.4,32.13 42.55,33.27 42.55,38.61 43.18,39.24 43.18,42.55 | v43.69,42.67 43.31,42.67 43.18,42.55
SDA_INTERNAL  (via drill 0.2)
  Top 0.203: U11.57 33.91,31.75 33.27,31.12 33.27,29.72 34.16,28.83 41.78,28.83 42.16,29.21 43.18,29.21 43.56,28.83 44.45,28.83 v44.7,29.08 | v44.45,47.37 42.67,47.37 42.55,47.24 38.1,47.24 38.03,47.32 R12.2 38.53,48.14 38.61,48.14 38.74,48.26 38.74,49.26 U7.19
  Bottom 0.203: v44.45,47.37 46.1,45.72 46.1,42.93 46.99,42.04 46.99,40.13 45.72,38.86 45.72,32.89 44.83,32 44.83,29.21 v44.7,29.08
USB_D+  (via drill 0.2, 0.2 pad 0.41)
  Top 0.203: U11.63 36.91,31.8 v37.08,31.62 | TP4.TP 26.67,45.97 v27.18,45.59
  Bottom 0.203: v37.08,31.62 37.08,38.23 36.7,38.61 27.18,38.61 26.42,39.37 26.42,40.89 26.8,41.27 26.8,43.56 27.18,43.81 v27.18,45.59 27.18,45.97 26.67,46.48 25.4,46.48 24.64,47.24 24.64,49.15 24.38,49.4 24.38,57.4 24.51,57.53 29.34,57.53 29.46,57.66 29.46,58.55 30.23,59.31 30.23,60.96 J1.11
USB_D-  (via drill 0.2, 0.2 pad 0.41)
  Top 0.203: U11.62 36.41,32.3 36.45,32.13 v36.45,30.99 | TP5.TP 25.02,46.36 v25.53,45.72
  Bottom 0.203: v36.45,30.99 36.45,37.97 36.2,38.23 26.54,38.23 26.42,38.35 26.42,38.86 26.04,39.24 26.04,41.02 26.42,41.4 26.42,43.69 26.67,43.94 26.67,45.85 26.42,46.1 25.53,46.1 | 25.53,46.1 25.15,46.1 24.26,46.99 24.26,49.02 24,49.28 24,57.91 24.26,58.17 28.7,58.17 28.96,58.42 J1.12 | v25.53,45.72 25.53,46.1
V_GSM_INT
  Top 0.203: U12.P$4 21.64,26.72 21.97,27.05 | 21.97,27.05 21.97,28.19 22.22,28.45 23.35,28.45 U10.2 | R10.2 27.94,27.81 26.29,26.16 22.1,26.16 21.97,26.29 21.97,27.05

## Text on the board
tNames: GND | 5V | 3V8 | 3V3 | GSM / GPIO2 | Aux / UART | USB+ | USB- | IN | OUT | PPS | RTS | CTS | GSM | RST | RX | PWR | GSM | TX | Joshua Adkins | Signpost Radio Module | 09/2016 | Rev_A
